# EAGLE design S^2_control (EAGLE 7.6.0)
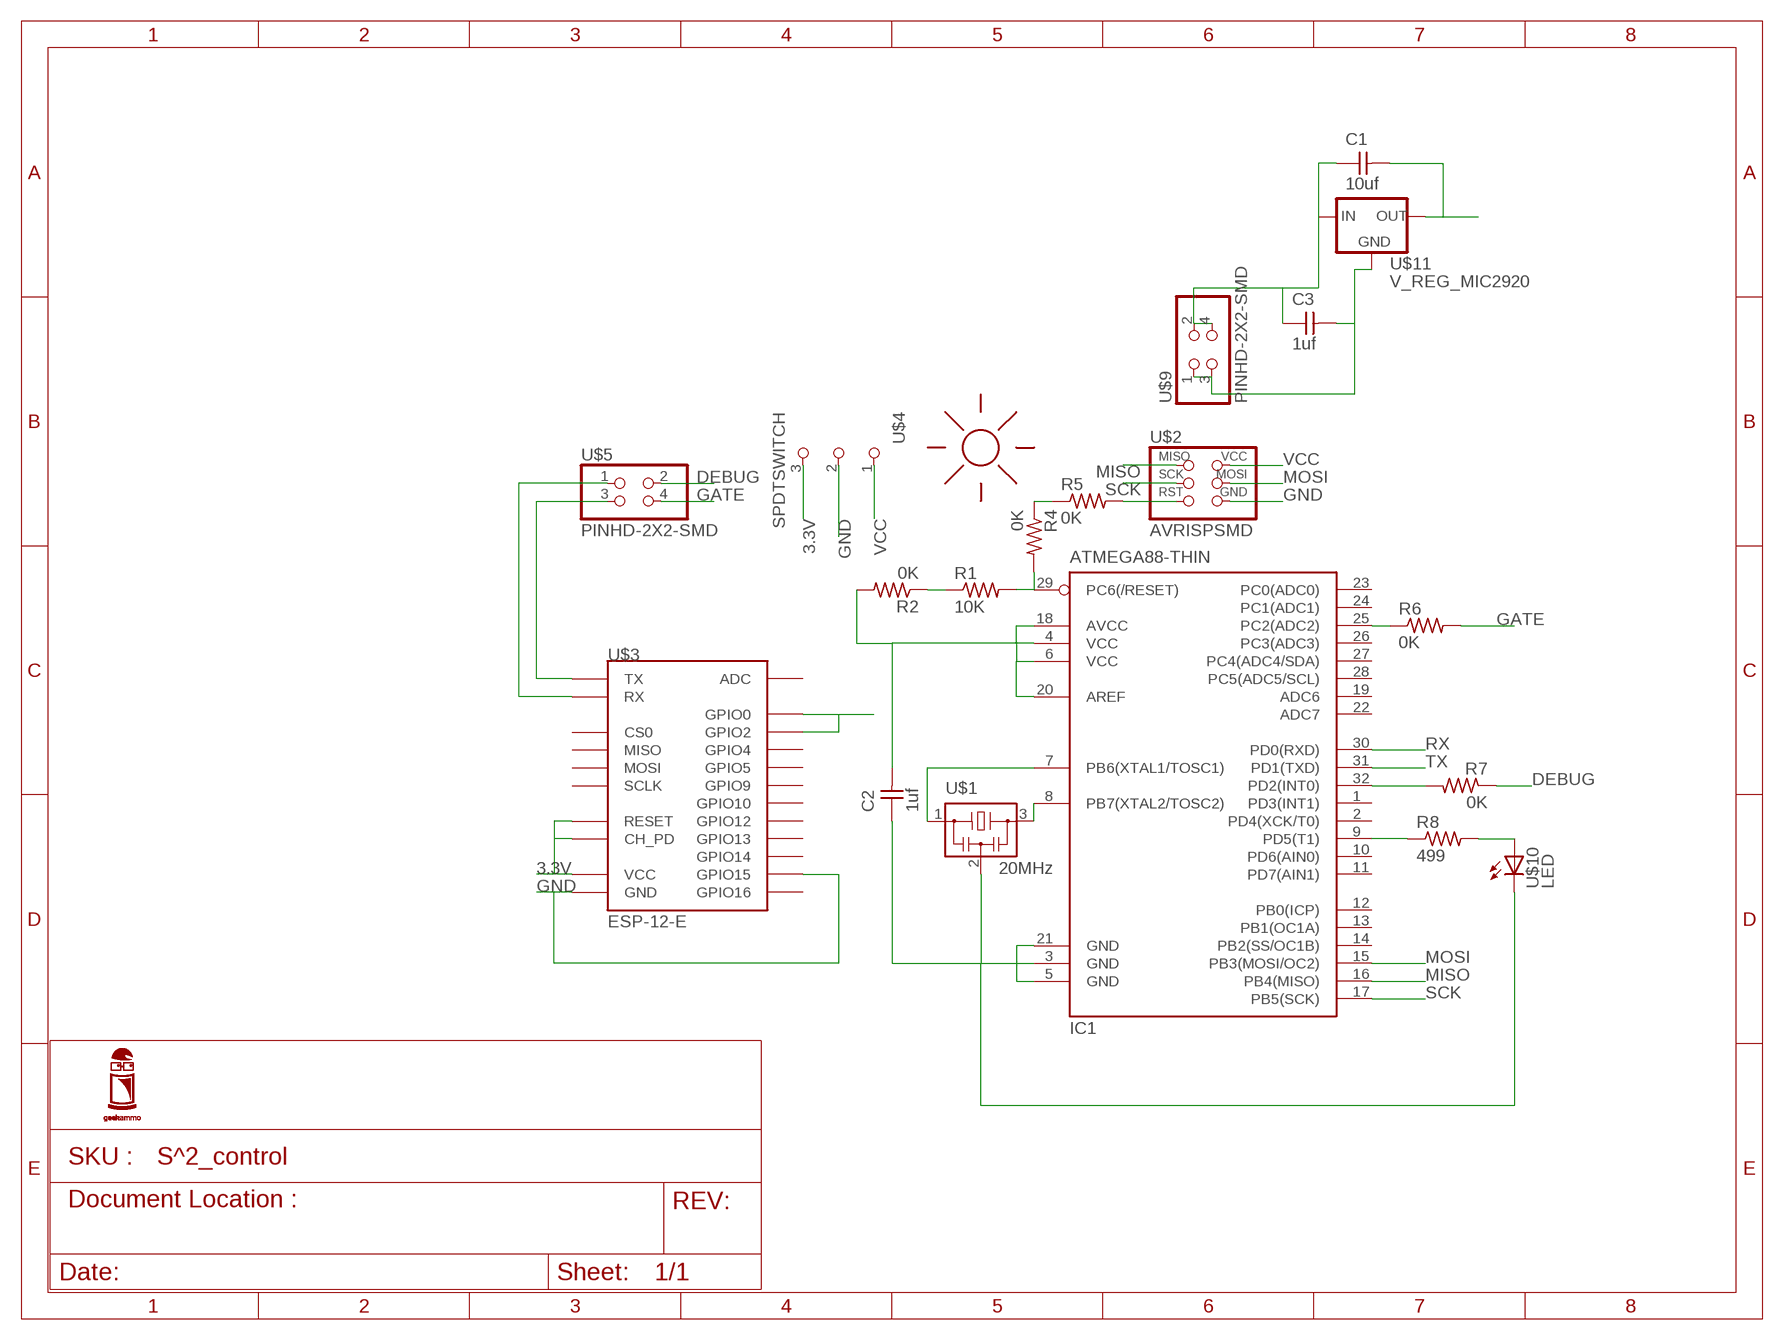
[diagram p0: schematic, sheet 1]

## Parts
C1  10uf  CAP-UNPOLARIZEDFAB  [C1206FAB]
C2  1uf  CAP-UNPOLARIZEDFAB  [C1206FAB]
C3  1uf  CAP-UNPOLARIZEDFAB  [C1206FAB]
IC1  ATMEGA88-THIN  [TQFP32-08THIN]
R1  10K  RES-US1206FAB  [R1206FAB]
R2  0K  RES-US1206FAB  [R1206FAB]
R4  0K  RES-US1206FAB  [R1206FAB]
R5  0K  RES-US1206FAB  [R1206FAB]
R6  0K  RES-US1206FAB  [R1206FAB]
R7  0K  RES-US1206FAB  [R1206FAB]
R8  499  RES-US1206FAB  [R1206FAB]
U$1  20MHz  RESONATOR  [EFOBM]
U$2  AVRISPSMD  [2X03SMD]
U$3  ESP-12-E  [ESP-12-E]
U$4  SPDTSWITCH  [SPDTSWITCH]
U$5  PINHD-2X2-SMD  [2X02SMD]
U$6  SUNLOGO  [SUN]
U$9  PINHD-2X2-SMD  [2X02SMD]
U$10  LED  LEDFAB1206  [LED1206FAB]
U$11  V_REG_MIC2920  [SOT223]

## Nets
3.3V: U$3.CH_PD U$3.GPIO0 U$3.GPIO2 U$3.RESET U$3.VCC U$4.3
DEBUG: R7.1 U$5.2
GATE: R6.2 U$5.4
GND: C2.1 C3.2 IC1.3(GND) IC1.5(GND) IC1.21(GND) U$1.2 U$2.6(GND) U$3.GND U$3.GPIO15 U$4.2 U$9.1 U$9.3 U$10.2(C) U$11.2(GND)
MISO: IC1.16(PB4(MISO)) U$2.1(MISO)
MOSI: IC1.15(PB3(MOSI/OC2)) U$2.4(MOSI)
N$1: IC1.32(PD2(INT0)) R7.2
N$2: IC1.9(PD5(T1)) R8.1
N$4: IC1.8(PB7(XTAL2/TOSC2)) U$1.3
N$5: IC1.7(PB6(XTAL1/TOSC1)) U$1.1
N$7: R8.2 U$10.1(A)
N$8: R1.1 R2.1
N$9: R5.2 U$2.5(RST)
N$10: R4.1 R5.1
N$11: IC1.25(PC2(ADC2)) R6.1
N$12: C1.1 C3.1 U$9.2 U$9.4 U$11.1(IN)
RST: IC1.29(PC6(/RESET)) R1.2 R4.2
RX: IC1.30(PD0(RXD)) U$3.TX U$5.3
SCK: IC1.17(PB5(SCK)) U$2.3(SCK)
TX: IC1.31(PD1(TXD)) U$3.RX U$5.1
VCC: C1.2 C2.2 IC1.4(VCC) IC1.6(VCC) IC1.18(AVCC) IC1.20(AREF) R2.2 U$2.2(VCC) U$4.1 U$11.3(OUT)
Unconnected: IC1.1(PD3(INT1)) IC1.2(PD4(XCK/T0)) IC1.10(PD6(AIN0)) IC1.11(PD7(AIN1)) IC1.12(PB0(ICP)) IC1.13(PB1(OC1A)) IC1.14(PB2(SS/OC1B)) IC1.19(ADC6) IC1.22(ADC7) IC1.23(PC0(ADC0)) IC1.24(PC1(ADC1)) IC1.26(PC3(ADC3)) IC1.27(PC4(ADC4/SDA)) IC1.28(PC5(ADC5/SCL)) U$3.ADC U$3.CS0 U$3.GPIO4 U$3.GPIO5 U$3.GPIO9 U$3.GPIO10 U$3.GPIO12 U$3.GPIO13 U$3.GPIO14 U$3.GPIO16 U$3.MISO U$3.MOSI U$3.SCLK

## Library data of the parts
C1-C3 = fab:CAP-UNPOLARIZED
IC1 = fab:ATMEGA88-THIN
R1 R2 R4-R8 = fab:RES-US: Resistor (US Symbol)
U$1 = fab:RESONATOR
U$2 = fab:AVRISP
U$3 = esp8266modules:ESP-12-E: ESP8266 Wifi Module ESP-12-E; DIMENSIONS: 24.0 x 16.0 mm; PINS: 22; PITCH: 0.078" / 2 mm
U$4 = fab:SPDTSWITCH
U$5 U$9 = fab:PINHD-2X2-SMD
U$6 = adafruit:SUNLOGO: Just a SMT logo of a sun. cute!
U$10 = fab:LED: LED
U$11 = SparkFun-PowerIC:V_REG_MIC2920: MIC2920A (http://www.micrel.com/_PDF/mic2920.pdf) - 400mA output LDO Regulator

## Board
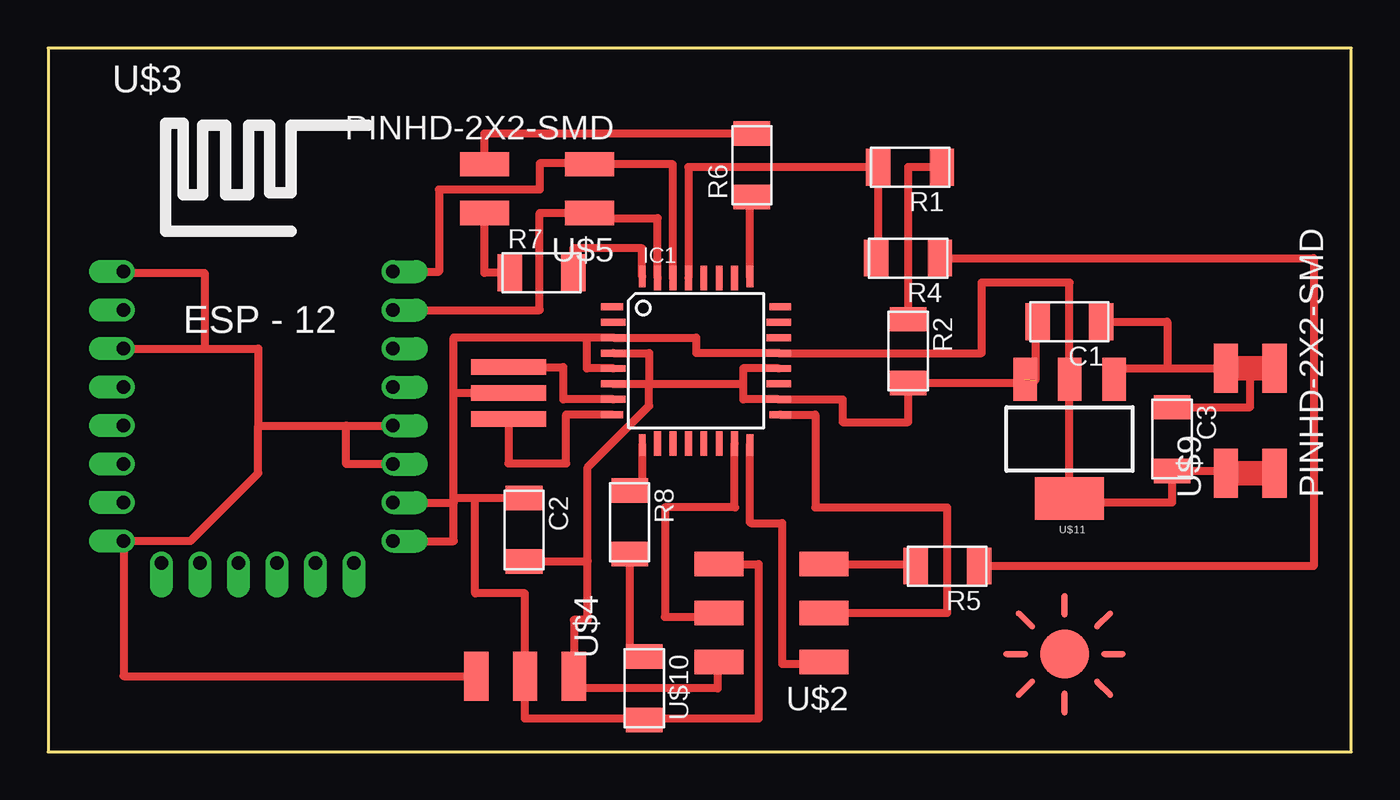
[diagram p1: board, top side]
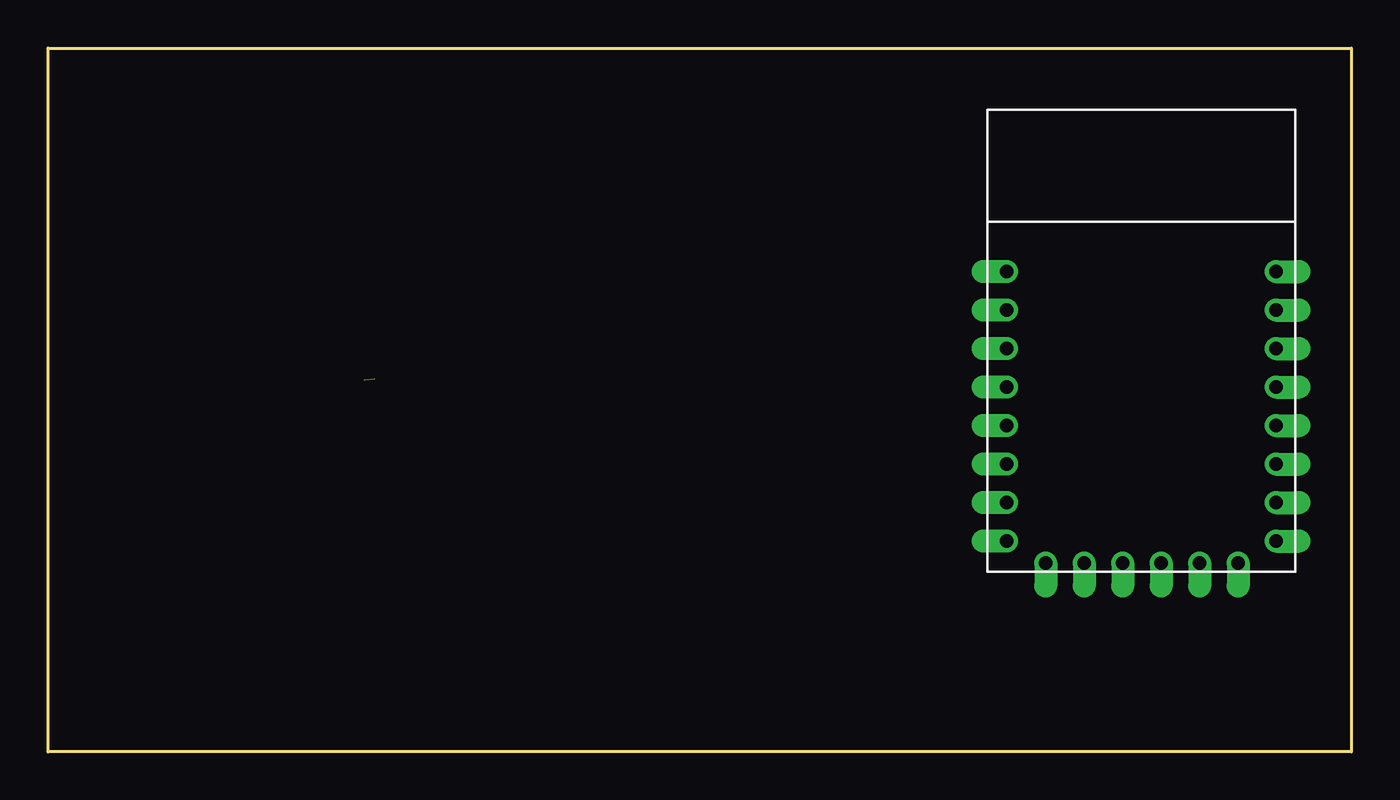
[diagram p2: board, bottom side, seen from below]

Size 67.74 x 36.57 mm. Coordinates in mm from the lower left corner, seen from the top.
Outline: 0,0 67.74,0 67.74,36.57 0,36.57 0,0
Copper layers (1*16): Top 0.035mm / dielectric 1.5mm / Bottom 0.035mm
Design rules "default *": minimum track width 16mil, minimum drill 24mil, track to track 16mil, track to pad 16mil, pad to pad 8mil, via to via 8mil, smd to smd 8mil, copper to edge 40mil, drill to drill 16mil, minimum pad ring 10mil, minimum via ring 8mil, stop-mask expansion 4mil, vias tented up to drill 0mil, thermal gap 10mil

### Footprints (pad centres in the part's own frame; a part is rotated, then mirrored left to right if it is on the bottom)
C1206FAB = smd 1.27 x 1.905: 1 -1.651,0; 2 1.651,0
TQFP32-08THIN = smd 1.118 x 0.356: 1 -4.369,2.8; 8 -4.369,-2.8; 17 4.369,-2.8; 24 4.369,2.8 | smd 1.27 x 0.356: 2 -4.293,2; 3 -4.293,1.2; 4 -4.293,0.4; 5 -4.293,-0.4; 6 -4.293,-1.2; 7 -4.293,-2; 18 4.293,-2; 19 4.293,-1.2; 20 4.293,-0.4; 21 4.293,0.4; 22 4.293,1.2; 23 4.293,2 | smd 0.356 x 1.118: 9 -2.8,-4.369; 16 2.8,-4.369; 25 2.8,4.369; 32 -2.8,4.369 | smd 0.356 x 1.27: 10 -2,-4.293; 14 1.2,-4.293; 15 2,-4.293; 26 2,4.293; 27 1.2,4.293; 31 -2,4.293 | smd 0.35 x 1.27: 11 -1.2,-4.293; 12 -0.4,-4.293; 13 0.4,-4.293; 28 0.4,4.293; 29 -0.4,4.293; 30 -1.2,4.293
R1206FAB = smd 1.27 x 1.905: 1 -1.651,0; 2 1.651,0
EFOBM = smd 0.8 x 3.9: 1 -1.35,0; 2 0,0; 3 1.35,0
2X03SMD = smd 2.54 x 1.27: 1 -2.54,2.54; 2 2.92,2.54; 3 -2.54,0; 4 2.92,0; 5 -2.54,-2.54; 6 2.92,-2.54
ESP-12-E = drill 0.7 offset: ADC -7.1,3.8; CH_PD -7.1,1.8; CS0 -5.14,-9.33; GND 6.9,-8.2; GPIO0 6.9,-2.2; GPIO2 6.9,-4.2; GPIO4 6.9,1.8; GPIO5 6.9,-0.2; GPIO9 -1.14,-9.33; GPIO10 0.86,-9.33; GPIO12 -7.1,-4.2; GPIO13 -7.1,-6.2; GPIO14 -7.1,-2.2; GPIO15 6.9,-6.2; GPIO16 -7.1,-0.2; MISO -3.14,-9.33; MOSI 2.86,-9.33; RESET -7.1,5.8; RX 6.9,3.8; SCLK 4.86,-9.33; TX 6.9,5.8; VCC -7.1,-8.2
SPDTSWITCH = smd 2.54 x 1.27: 1 0.38,2.54; 2 0.38,0; 3 0.38,-2.54
2X02SMD = smd 2.54 x 1.27: 1 -2.54,1.27; 2 2.92,1.27; 3 -2.54,-1.27; 4 2.92,-1.27
SUN = smd 2.54 x 2.54: P$1 0,0 | smd 0.305 x 1.27: P$2 0,2.54; P$3 0,-2.54 | smd 1.27 x 0.305: P$4 2.54,0; P$5 -2.54,0 | smd 1.27 x 0.305 rotated 45: P$6 2.032,1.778 | smd 1.27 x 0.305 rotated 135: P$7 2.032,-1.778 | smd 1.27 x 0.305 rotated 225: P$8 -2.032,-1.778 | smd 1.27 x 0.305 rotated 315: P$9 -2.032,1.778
LED1206FAB = smd 1.27 x 1.905: 1 -1.651,0; 2 1.651,0
SOT223 = smd 1.219 x 2.235: 1 -2.311,-3.099; 2 0,-3.099; 3 2.311,-3.099 | smd 3.6 x 2.2: 4 0,3.099

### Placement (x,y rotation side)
C1  53.09,22.35 180 top
C2  24.74,11.53 270 top
C3  58.42,16.26 270 top
IC1  33.68,20.32 0 top
R1  44.81,30.38 180 top
R2  44.7,20.83 270 top
R4  44.7,25.65 180 top
R5  46.74,9.65 180 top
R6  36.58,30.48 90 top
R7  25.65,24.89 0 top
R8  30.23,11.94 270 top
U$1  23.93,18.64 270 top
U$2  37.8,7.21 180 top
U$3  11.02,19.15 0 top
U$4  24.79,4.32 270 top
U$5  25.6,29.26 180 top
U$6  52.83,5.08 0 top
U$9  62.48,17.02 90 top
U$10  30.99,3.3 270 top
U$11  53.09,16.26 180 top

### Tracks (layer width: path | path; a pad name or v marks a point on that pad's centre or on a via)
3.3V
  Top 0.406: U$4.3 3.92,3.94 U$3.VCC 7.4,10.95 10.92,14.48 10.92,16.95 | U$3.CH_PD 8.13,20.95 | 8.13,20.95 10.92,20.95 10.92,16.95 | U$3.RESET 3.92,24.89 8.13,24.89 8.13,20.95 | 10.92,16.95 15.49,16.95 | 15.49,16.95 U$3.GPIO0 | U$3.GPIO2 15.49,14.95 15.49,16.95
DEBUG
  Top 0.406: R7.1 22.68,24.89 U$5.2
GATE
  Top 0.406: U$5.4 22.68,32.13 R6.2
GND
  Top 0.406: 27.99,21.52 IC1.3 33.68,21.52 33.68,20.72 IC1.21 48.51,20.72 48.51,24.38 53.09,24.38 U$11.2 53.09,12.95 58.42,12.95 C3.2 61.72,14.61 61.72,14.48 | 27.99,21.52 27.99,19.92 IC1.5 | C2.1 22.2,13.18 | 22.2,13.18 21.08,13.18 | 21.08,13.18 21.08,18.64 | U$1.2 21.08,18.64 | 21.08,18.64 21.08,21.52 27.99,21.52 | 22.2,13.18 22.2,8.23 24.79,8.23 U$4.2 24.79,1.73 30.99,1.73 | U$2.6 36.93,9.75 36.93,1.73 30.99,1.73 | U$3.GND 21.08,10.95 21.08,12.95 | 21.08,12.95 21.08,13.18 | U$10.2 30.99,1.73 | U$3.GPIO15 21.08,12.95
  Top 1.27: U$9.1 61.72,14.48 U$9.3
MISO
  Top 0.406: U$2.1 40.34,4.57 38.15,4.57 38.15,11.89 36.52,11.89 36.48,11.93 IC1.16
MOSI
  Top 0.406: U$2.4 34.88,7.01 32.05,7.01 32.05,12.7 35.71,12.7 35.68,12.73 IC1.15
N$1
  Top 0.406: IC1.32 30.88,26.16 27.3,26.16 R7.2
N$2
  Top 0.406: IC1.9 30.88,13.59 R8.1
N$4
  Top 0.406: IC1.8 26.92,17.52 26.92,14.99 23.93,14.99 U$1.3
N$5
  Top 0.406: U$1.1 26.77,19.99 26.77,18.32 IC1.7
N$7
  Top 0.406: R8.2 30.23,4.95 U$10.1
N$8
  Top 0.406: R1.1 44.7,30.38 R2.1
N$9
  Top 0.406: U$2.5 45.09,9.75 R5.2
N$10
  Top 0.406: R4.1 65.79,25.65 65.79,9.65 R5.1
N$11
  Top 0.406: IC1.25 36.48,28.83 R6.1
N$12
  Top 0.406: U$11.1 55.4,19.94 58.17,19.94 | 58.17,19.94 62.23,19.94 | C3.1 62.48,17.91 62.48,19.94 | C1.1 58.17,22.35 58.17,19.94
  Top 1.27: U$9.4 62.48,19.94 62.23,19.94 U$9.2
RST
  Top 0.406: R4.2 43.16,25.65 R1.2 33.27,30.38 IC1.29
RX
  Top 0.406: IC1.30 32.48,30.53 U$5.3 28.14,30.58 25.55,30.58 25.55,29.21 20.32,29.21 20.32,24.95 U$3.TX
SCK
  Top 0.406: U$2.3 46.74,7.21 46.74,12.7 39.88,12.7 39.88,17.52 IC1.17
TX
  Top 0.406: IC1.31 31.68,27.74 28.14,27.74 U$5.1 25.55,27.99 25.55,22.95 U$3.RX
VCC  (1 unrouted)
  Top 0.406: IC1.4 31.24,20.72 31.24,19.12 | IC1.6 31.24,19.12 | IC1.20 36.12,19.92 36.12,19.12 | 36.12,19.12 36.12,18.32 IC1.18 41.3,18.32 41.3,17.14 44.7,17.14 R2.2 50.77,19.18 U$11.3 | 28.04,9.91 28.04,6.86 27.33,6.86 U$4.1 27.33,3.3 34.8,3.3 34.8,4.67 U$2.2 | 28.04,9.91 28.04,14.78 31.24,17.98 31.24,19.12 | 31.24,19.12 36.12,19.12 | C2.2 24.74,9.91 28.04,9.91 | C1.2 51.31,22.35 51.31,19.3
